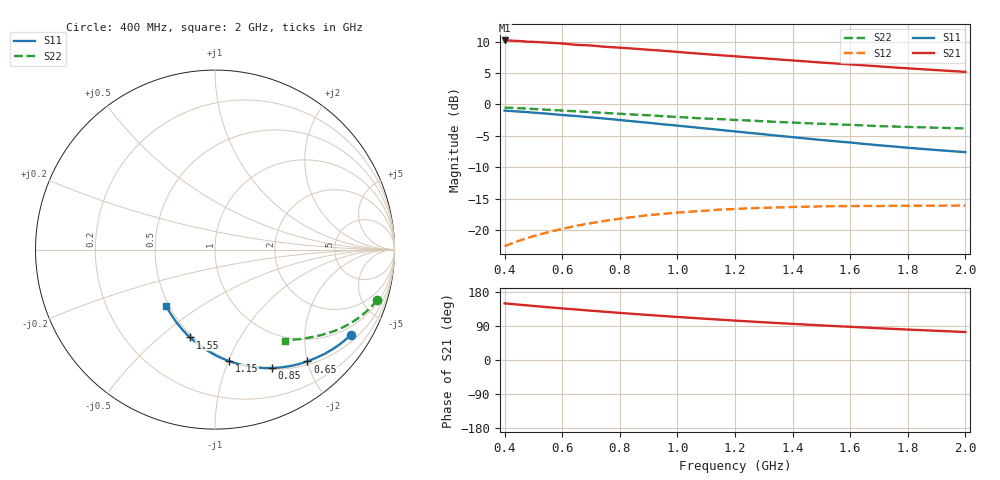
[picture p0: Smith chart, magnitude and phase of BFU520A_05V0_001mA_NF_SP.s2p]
! Filename:  P:\Prog\Test\Noise\ATS_data\Testdata_Net\06 Compressed Noise after Statistics\BFU520A_APG2013_30_A05_05p0V_001mA_NF_CM01_D.sf
! Date/Time: Wed 24/Apr/2013 20:06:17
! BFU520A_APG2013_30_A05_05p0V_1to20mA_NF_CM01_Bias1_R.sf
! Noise Parameter Data File
! BFU520A_APG2013_30_A05_05p0V_1to20mA_NF_CM01
! Date/time: Thu Apr 11 01:07:08 2013
! freq range =  0.4000 to  2.0000 GHz, 37 points
! bias range =  1.0000 to 19.9950 mA, 8 points
! bias supplies used: 1 1 0 0 0 0
! VAR bias_mode= 1  ! Specify V_out, I_out
! VAR bias_var = 1  ! Bias variable = I_out
! VAR V_out= 5.001000
! VAR I_out= 1.000000
! VAR V_in= 0.793000
! VAR I_in= 0.010600
! Device data file deembeded for feedlines and parallel
! Original file: \06 Compressed Noise after Statistics\BFU520A_APG2013_30_A05_05p0V_001mA_NF_CM01_R.sf
! Feed-files: PR017V01_150413_Feed1.s2p, PR017V01_150413_Feed2.s2p
! Parallel-file: PR017V01_150413_Par.s2p
# MHz S MA R 50
!  Freq-MHz  S11-mag  S11-arg  S21-mag  S21-arg  S12-mag  S12-arg  S22-mag  S22-arg
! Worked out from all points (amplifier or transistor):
!   37 points, 400 MHz to 2 GHz, reference 50 ohm
!   highest |S21| = 10.2 dB at 400 MHz (marker M1)
!   |S21| within 3 dB of that: start of sweep to 1.343 GHz
!   unconditionally stable (mu >= 1): nowhere
!   at 500 MHz: K = 0.23, MSG = 15.5 dB, |S12| = -21.0 dB
!   at 1.1 GHz: K = 0.49, MSG = 12.5 dB, |S12| = -16.9 dB
!   at 2 GHz: K = 0.87, MSG = 10.7 dB, |S12| = -16.1 dB
!   lowest NFmin = 0.50 dB at 420 MHz
!   S11 on the Smith chart (normalised r, x): 400 MHz: 0.71, -3.33; 650 MHz: 0.56, -2.00; 850 MHz: 0.52, -1.47; 1.15 GHz: 0.49, -1.00; 1.55 GHz: 0.48, -0.64; 2 GHz: 0.48, -0.37
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400  0.8934 -32.1  3.237 149.5  0.07418 69.4  0.9448 -17.3
440  0.8808 -35.3  3.213 146.7  0.08041 67.6  0.9358 -18.8
460  0.8743 -36.8  3.195 145.4  0.08339 66.7  0.9315 -19.5
480  0.8683 -38.2  3.161 144.0  0.08625 65.8  0.9256 -20.3
500  0.8608 -39.8  3.155 142.7  0.08909 65.0  0.9209 -21.0
550  0.8436 -43.5  3.111 139.4  0.0957 62.9  0.9072 -22.7
600  0.8241 -47.2  3.062 136.2  0.1019 61.0  0.8943 -24.4
650  0.8082 -50.5  2.986 133.2  0.1079 59.2  0.8815 -25.9
700  0.7893 -54.1  2.951 130.1  0.1132 57.5  0.868 -27.5
750  0.7711 -57.4  2.88 127.2  0.1182 55.8  0.8556 -28.9
800  0.7518 -60.9  2.836 124.3  0.1228 54.2  0.8427 -30.3
850  0.7323 -64.2  2.784 121.5  0.127 52.7  0.8306 -31.6
950  0.6948 -70.7  2.681 116.1  0.1341 50.0  0.8059 -34.1
1050  0.6604 -76.8  2.568 111.1  0.1399 47.8  0.7823 -36.4
1150  0.6262 -82.9  2.467 106.3  0.1452 45.7  0.7637 -38.4
1200  0.6096 -85.9  2.422 104.0  0.1467 44.8  0.7523 -39.5
1350  0.5628 -94.6  2.285 97.4  0.151 42.7  0.7248 -42.3
1500  0.5209 -103.0  2.158 91.3  0.1539 41.1  0.7014 -44.8
1550  0.5086 -105.8  2.121 89.4  0.1547 40.8  0.695 -45.7
1750  0.4624 -117.0  1.974 82.1  0.1556 40.3  0.6674 -48.8
1850  0.4425 -122.3  1.909 78.7  0.1561 40.3  0.6578 -50.3
2000  0.4166 -130.6  1.82 73.9  0.1565 41.3  0.6435 -52.5
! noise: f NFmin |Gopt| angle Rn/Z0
400  0.5249  0.6999  16.79  0.3554
460  0.5385  0.6794  21.38  0.3737
600  0.6179  0.6338  25.66  0.3631
800  0.579  0.6296  39.82  0.2842
1000  0.6131  0.6234  49.17  0.2697
1200  0.72  0.6063  58.49  0.2708
1400  0.7677  0.5873  69.37  0.23
1600  0.807  0.5399  79.36  0.1869
1800  0.6801  0.5315  93.33  0.1357
2000  0.8197  0.4946  101.4  0.1417
